(* Logix 5000 AddOnInstructionDefinition export Banner_R95C_MDR_PD_v5; software revision 33.00 *)

TYPE Banner_R95C_MDR_PDI_v5 :
STRUCT
   MDR_Short_Circuit : BOOL[32];   // 0=Inactive, 1=Active. Only 1 through 4 used.
   MDR_Overcurrent : BOOL[32];   // 0=Current Below Limit, 1=Current Above Limit. Only 1 through 4 used.
   MDR_OverVoltage : BOOL;   // 0=Voltage within Range, 1=Voltage above Range
   MDR_UnderVoltage : BOOL;   // 0=Voltage within Range, 1=Voltage below Range
   Block_Temperature : BOOL;   // 0=Temp below limit, 1=Temp above limit
   Aux_Power : BOOL;   // 0=No Aux Power, 1=Aux Power Present
   Port_Channel_1 : BOOL[32];   // 0=Off, 1=On. Only 1 through 4 used.
   Port_Channel_2 : BOOL[32];   // 0=Off, 1=On. Only 1 through 4 used.
   Analog_Value : INT[5];
END_STRUCT
END_TYPE

TYPE Banner_R95C_MDR_PDIO_v5 :
STRUCT
   PDI : Banner_R95C_MDR_PDI_v5;
   PDO : Banner_R95C_MDR_PDO_v5;
   DTI : SINT[12];
   DTO : SINT[10];
END_STRUCT
END_TYPE

TYPE Banner_R95C_MDR_PDO_v5 :
STRUCT
   Motor_Current_Fault_Reset : BOOL[32];   // 0=No Action, 1=Reset. Only 1 through 4 used.
   Port_Channel_1_Control : BOOL[32];   // 0=Off, 1=On. Only 1 through 4 used.
   Port_Channel_2_Control : BOOL[32];   // 0=Off, 1=On. Only 1 through 4 used.
   Analog_Output : INT[5];
END_STRUCT
END_TYPE

ADD_ON_INSTRUCTION Banner_R95C_MDR_PDin_v5   (* revision 5.0 *)
VAR_INPUT
   Byte : SINT; {required}
END_VAR
VAR_OUTPUT
   Bool0 : BOOL; {required}
   Bool1 : BOOL; {required}
   Bool2 : BOOL; {required}
   Bool3 : BOOL; {required}
   Bool4 : BOOL; {required}
   Bool5 : BOOL; {required}
   Bool6 : BOOL; {required}
   Bool7 : BOOL; {required}
END_VAR

ROUTINE Logic   (* ladder *)
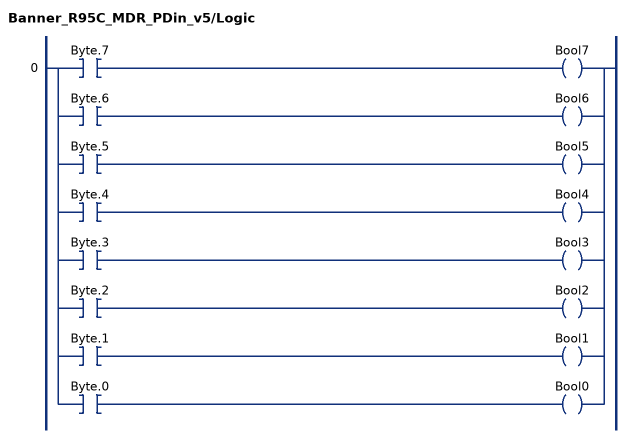
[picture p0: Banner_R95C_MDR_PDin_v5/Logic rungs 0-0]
   0: [XIC(Byte.7) OTE(Bool7) ,XIC(Byte.6) OTE(Bool6) ,XIC(Byte.5) OTE(Bool5) ,XIC(Byte.4) OTE(Bool4) ,XIC(Byte.3) OTE(Bool3) ,XIC(Byte.2) OTE(Bool2) ,XIC(Byte.1) OTE(Bool1) ,XIC(Byte.0) OTE(Bool0) ];
END_ROUTINE
END_ADD_ON_INSTRUCTION

ADD_ON_INSTRUCTION Banner_R95C_MDR_PD_v5   (* revision 5.0, vendor Banner Engineering *)
// AOI that used with the R95C-L-4MDR-KQ hub.
VAR_IN_OUT
   PD : Banner_R95C_MDR_PDIO_v5; {required}
END_VAR
VAR_INPUT
   Byte_Swap : BOOL; {required}
END_VAR
VAR
   TempIn : SINT[12]; {access None}
   TempOut : SINT[10]; {access None}
   Blank : BOOL[32]; {access None}
   Status : Banner_R95C_MDR_PDin_v5[3]; {access None}
END_VAR

ROUTINE Logic   (* ladder *)
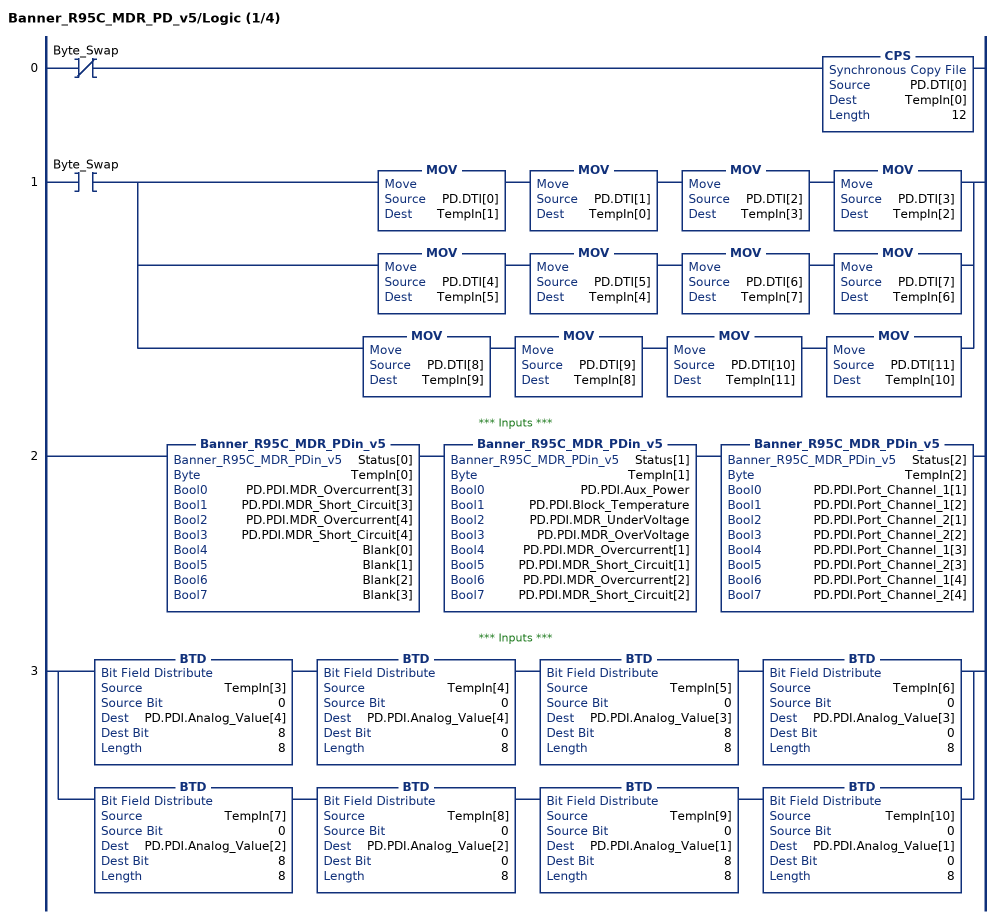
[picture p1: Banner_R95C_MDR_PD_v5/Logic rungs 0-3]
   0: XIO(Byte_Swap)CPS(PD.DTI[0],TempIn[0],12);
   1: XIC(Byte_Swap)[MOV(PD.DTI[0],TempIn[1]) MOV(PD.DTI[1],TempIn[0]) MOV(PD.DTI[2],TempIn[3]) MOV(PD.DTI[3],TempIn[2]) ,MOV(PD.DTI[4],TempIn[5]) MOV(PD.DTI[5],TempIn[4]) MOV(PD.DTI[6],TempIn[7]) MOV(PD.DTI[7],TempIn[6]) ,MOV(PD.DTI[8],TempIn[9]) MOV(PD.DTI[9],TempIn[8]) MOV(PD.DTI[10],TempIn[11]) MOV(PD.DTI[11],TempIn[10]) ];
   // *** Inputs ***
   2: Banner_R95C_MDR_PDin_v5(Status[0],TempIn[0],PD.PDI.MDR_Overcurrent[3],PD.PDI.MDR_Short_Circuit[3],PD.PDI.MDR_Overcurrent[4],PD.PDI.MDR_Short_Circuit[4],Blank[0],Blank[1],Blank[2],Blank[3])Banner_R95C_MDR_PDin_v5(Status[1],TempIn[1],PD.PDI.Aux_Power,PD.PDI.Block_Temperature,PD.PDI.MDR_UnderVoltage,PD.PDI.MDR_OverVoltage,PD.PDI.MDR_Overcurrent[1],PD.PDI.MDR_Short_Circuit[1],PD.PDI.MDR_Overcurrent[2],PD.PDI.MDR_Short_Circuit[2])Banner_R95C_MDR_PDin_v5(Status[2],TempIn[2],PD.PDI.Port_Channel_1[1],PD.PDI.Port_Channel_1[2],PD.PDI.Port_Channel_2[1],PD.PDI.Port_Channel_2[2],PD.PDI.Port_Channel_1[3],PD.PDI.Port_Channel_2[3],PD.PDI.Port_Channel_1[4],PD.PDI.Port_Channel_2[4]);
   // *** Inputs ***
   3: [BTD(TempIn[3],0,PD.PDI.Analog_Value[4],8,8) BTD(TempIn[4],0,PD.PDI.Analog_Value[4],0,8) BTD(TempIn[5],0,PD.PDI.Analog_Value[3],8,8) BTD(TempIn[6],0,PD.PDI.Analog_Value[3],0,8) ,BTD(TempIn[7],0,PD.PDI.Analog_Value[2],8,8) BTD(TempIn[8],0,PD.PDI.Analog_Value[2],0,8) BTD(TempIn[9],0,PD.PDI.Analog_Value[1],8,8) BTD(TempIn[10],0,PD.PDI.Analog_Value[1],0,8) ];
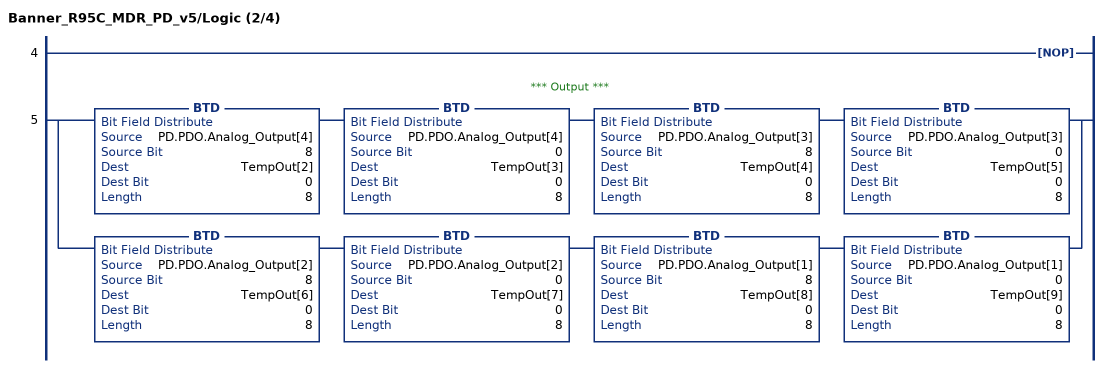
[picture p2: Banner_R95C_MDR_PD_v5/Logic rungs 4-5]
   4: NOP();
   // *** Output ***
   5: [BTD(PD.PDO.Analog_Output[4],8,TempOut[2],0,8) BTD(PD.PDO.Analog_Output[4],0,TempOut[3],0,8) BTD(PD.PDO.Analog_Output[3],8,TempOut[4],0,8) BTD(PD.PDO.Analog_Output[3],0,TempOut[5],0,8) ,BTD(PD.PDO.Analog_Output[2],8,TempOut[6],0,8) BTD(PD.PDO.Analog_Output[2],0,TempOut[7],0,8) BTD(PD.PDO.Analog_Output[1],8,TempOut[8],0,8) BTD(PD.PDO.Analog_Output[1],0,TempOut[9],0,8) ];
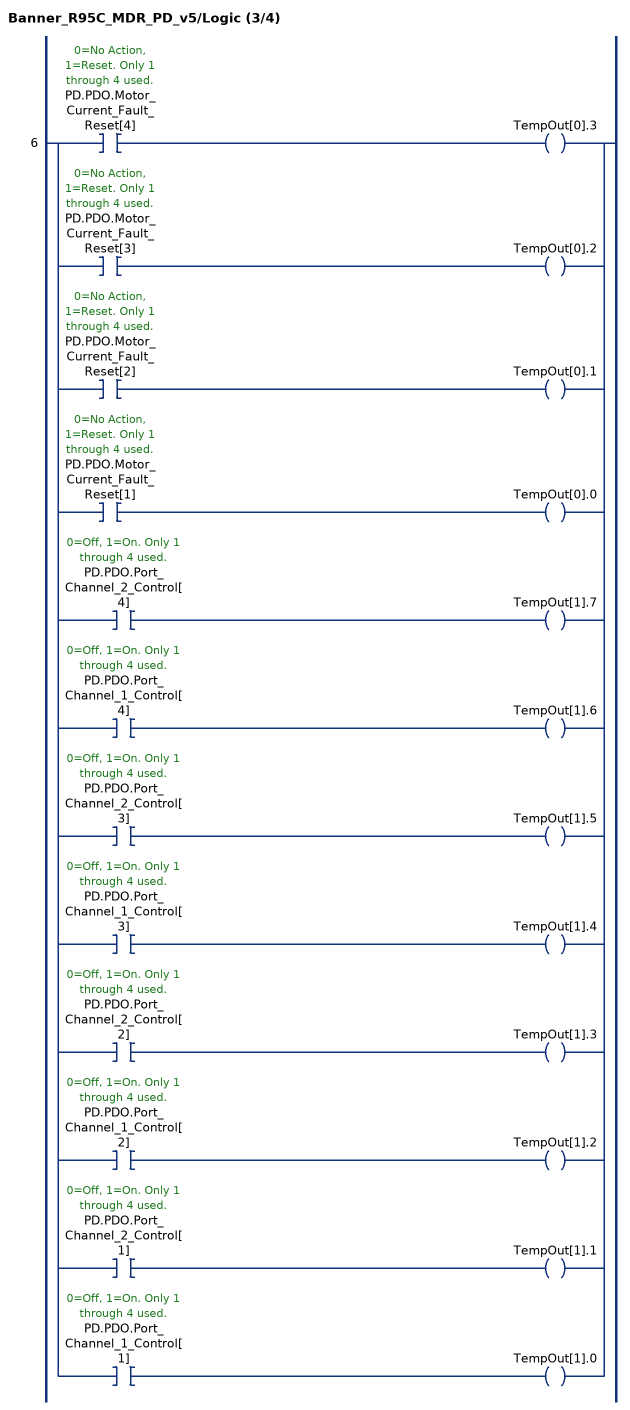
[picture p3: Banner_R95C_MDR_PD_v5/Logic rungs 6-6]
   6: [XIC(PD.PDO.Motor_Current_Fault_Reset[4]) OTE(TempOut[0].3) ,XIC(PD.PDO.Motor_Current_Fault_Reset[3]) OTE(TempOut[0].2) ,XIC(PD.PDO.Motor_Current_Fault_Reset[2]) OTE(TempOut[0].1) ,XIC(PD.PDO.Motor_Current_Fault_Reset[1]) OTE(TempOut[0].0) ,XIC(PD.PDO.Port_Channel_2_Control[4]) OTE(TempOut[1].7) ,XIC(PD.PDO.Port_Channel_1_Control[4]) OTE(TempOut[1].6) ,XIC(PD.PDO.Port_Channel_2_Control[3]) OTE(TempOut[1].5) ,XIC(PD.PDO.Port_Channel_1_Control[3]) OTE(TempOut[1].4) ,XIC(PD.PDO.Port_Channel_2_Control[2]) OTE(TempOut[1].3) ,XIC(PD.PDO.Port_Channel_1_Control[2]) OTE(TempOut[1].2) ,XIC(PD.PDO.Port_Channel_2_Control[1]) OTE(TempOut[1].1) ,XIC(PD.PDO.Port_Channel_1_Control[1]) OTE(TempOut[1].0) ];
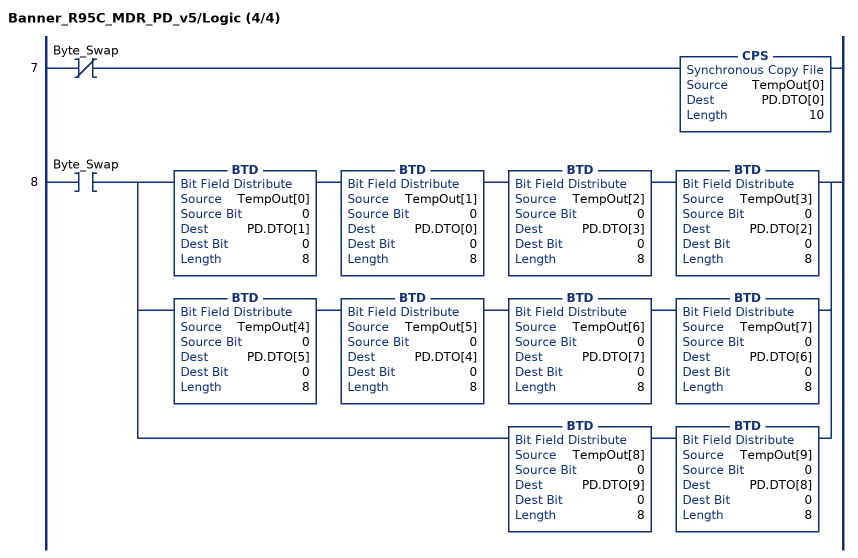
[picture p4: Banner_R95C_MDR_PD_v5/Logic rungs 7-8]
   7: XIO(Byte_Swap)CPS(TempOut[0],PD.DTO[0],10);
   8: XIC(Byte_Swap)[BTD(TempOut[0],0,PD.DTO[1],0,8) BTD(TempOut[1],0,PD.DTO[0],0,8) BTD(TempOut[2],0,PD.DTO[3],0,8) BTD(TempOut[3],0,PD.DTO[2],0,8) ,BTD(TempOut[4],0,PD.DTO[5],0,8) BTD(TempOut[5],0,PD.DTO[4],0,8) BTD(TempOut[6],0,PD.DTO[7],0,8) BTD(TempOut[7],0,PD.DTO[6],0,8) ,BTD(TempOut[8],0,PD.DTO[9],0,8) BTD(TempOut[9],0,PD.DTO[8],0,8) ];
END_ROUTINE
END_ADD_ON_INSTRUCTION
